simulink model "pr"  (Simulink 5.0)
settings: Solver=ode45  StartTime=0.0  StopTime=2  RelTol=1e-3
undefined symbols (not defined in the file or in its folder): sigbuilder_block
libraries: simulink x6

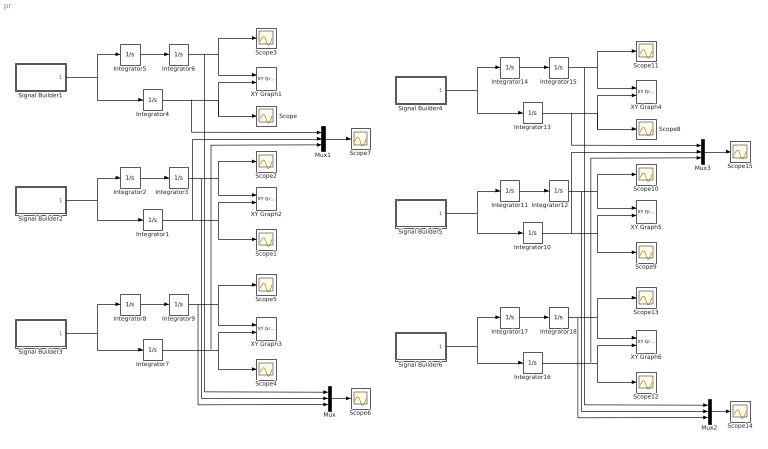
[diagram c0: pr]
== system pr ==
  Integrator{1..18} (18 alike) : Integrator
  Mux{,1..3} (4 alike) : Mux  Inputs=3
  Scope{,1..15} (16 alike) : Scope
  Signal Builder1 : Subsystem  Tag=STV Subsys  StartFcn=sigbuilder_block('start');  StopFcn=sigbuilder_block('stop');  ClipboardFcn=sigbuilder_block('clipboard');
  Signal Builder2 : Subsystem  Tag=STV Subsys  StartFcn=sigbuilder_block('start');  StopFcn=sigbuilder_block('stop');  ClipboardFcn=sigbuilder_block('clipboard');
  Signal Builder3 : Subsystem  Tag=STV Subsys  StartFcn=sigbuilder_block('start');  StopFcn=sigbuilder_block('stop');  ClipboardFcn=sigbuilder_block('clipboard');
  Signal Builder4 : Subsystem  Tag=STV Subsys  StartFcn=sigbuilder_block('start');  StopFcn=sigbuilder_block('stop');  ClipboardFcn=sigbuilder_block('clipboard');
  Signal Builder5 : Subsystem  Tag=STV Subsys  StartFcn=sigbuilder_block('start');  StopFcn=sigbuilder_block('stop');  ClipboardFcn=sigbuilder_block('clipboard');
  Signal Builder6 : Subsystem  Tag=STV Subsys  StartFcn=sigbuilder_block('start');  StopFcn=sigbuilder_block('stop');  ClipboardFcn=sigbuilder_block('clipboard');
  XY Graph1 : simulink/Sinks/XY Graph  xmin=0  xmax=3.5  ymin=0  ymax=3.5  st=-1
  XY Graph2 : simulink/Sinks/XY Graph  xmin=0  xmax=3.5  ymin=0  ymax=3.5  st=-1
  XY Graph3 : simulink/Sinks/XY Graph  xmin=0  xmax=3.5  ymin=0  ymax=3.5  st=-1
  XY Graph4 : simulink/Sinks/XY Graph  xmin=-4  xmax=0  ymin=-4  ymax=1.5  st=-1
  XY Graph5 : simulink/Sinks/XY Graph  xmin=-4  xmax=0  ymin=-4  ymax=1.5  st=-1
  XY Graph6 : simulink/Sinks/XY Graph  xmin=-4  xmax=0  ymin=-4  ymax=1.5  st=-1
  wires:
  Signal Builder1/1(Signal 2) -> Integrator4/1, Integrator5/1
  Integrator5/1 -> Integrator6/1
  Integrator6/1 -> XY Graph1/1, Scope3/1, Mux/1
  Integrator4/1 -> XY Graph1/2, Scope/1, Mux1/1
  Signal Builder2/1(Signal 2) -> Integrator1/1, Integrator2/1
  Integrator2/1 -> Integrator3/1
  Integrator3/1 -> XY Graph2/1, Scope2/1, Mux/2
  Integrator1/1 -> XY Graph2/2, Scope1/1, Mux1/2
  Signal Builder3/1(Signal 3) -> Integrator7/1, Integrator8/1
  Integrator8/1 -> Integrator9/1
  Integrator9/1 -> XY Graph3/1, Scope5/1, Mux/3
  Integrator7/1 -> XY Graph3/2, Scope4/1, Mux1/3
  Mux1/1 -> Scope7/1
  Mux/1 -> Scope6/1
  Signal Builder4/1(Signal 2) -> Integrator13/1, Integrator14/1
  Integrator14/1 -> Integrator15/1
  Integrator15/1 -> XY Graph4/1, Scope11/1, Mux2/1
  Integrator13/1 -> XY Graph4/2, Scope8/1, Mux3/1
  Signal Builder5/1(Signal 2) -> Integrator10/1, Integrator11/1
  Integrator11/1 -> Integrator12/1
  Integrator12/1 -> XY Graph5/1, Scope10/1, Mux2/2
  Integrator10/1 -> XY Graph5/2, Scope9/1, Mux3/2
  Signal Builder6/1(Signal 3) -> Integrator16/1, Integrator17/1
  Integrator17/1 -> Integrator18/1
  Integrator18/1 -> XY Graph6/1, Scope13/1, Mux2/3
  Integrator16/1 -> XY Graph6/2, Scope12/1, Mux3/3
  Mux3/1 -> Scope15/1
  Mux2/1 -> Scope14/1

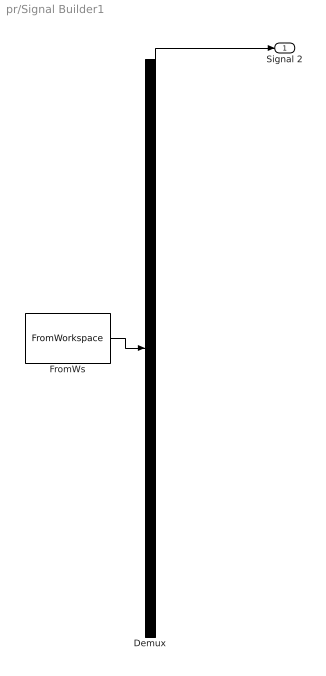
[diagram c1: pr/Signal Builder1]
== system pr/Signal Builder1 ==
  Demux : Demux  Tag=STV Demux  Outputs=1
  FromWs : FromWorkspace  Tag=STV FromWs  VariableName=tuvar  SampleTime=0  SigBuilderData=DataTag0
  Signal 2 : Outport  Tag=STV Outport
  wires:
  FromWs/1 -> Demux/1
  Demux/1 -> Signal 2/1

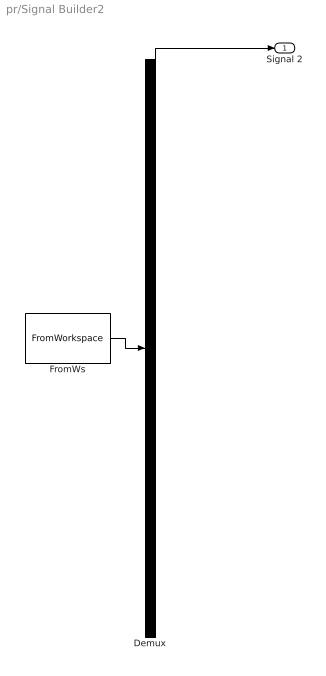
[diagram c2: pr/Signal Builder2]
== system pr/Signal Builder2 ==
  Demux : Demux  Tag=STV Demux  Outputs=1
  FromWs : FromWorkspace  Tag=STV FromWs  VariableName=tuvar  SampleTime=0  SigBuilderData=DataTag1
  Signal 2 : Outport  Tag=STV Outport
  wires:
  FromWs/1 -> Demux/1
  Demux/1 -> Signal 2/1

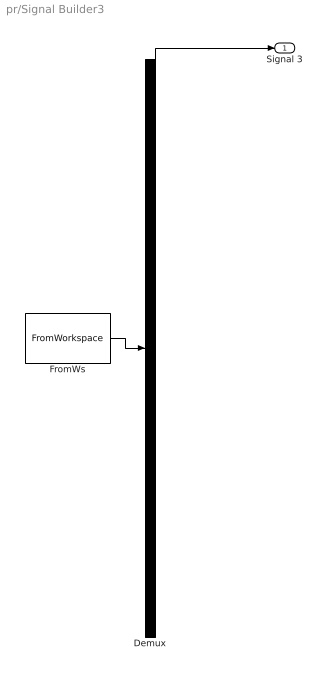
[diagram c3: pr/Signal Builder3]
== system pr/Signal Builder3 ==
  Demux : Demux  Tag=STV Demux  Outputs=1
  FromWs : FromWorkspace  Tag=STV FromWs  VariableName=tuvar  SampleTime=0  SigBuilderData=DataTag2
  Signal 3 : Outport  Tag=STV Outport
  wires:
  FromWs/1 -> Demux/1
  Demux/1 -> Signal 3/1

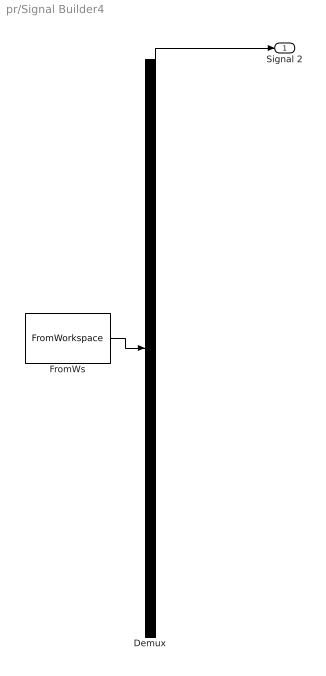
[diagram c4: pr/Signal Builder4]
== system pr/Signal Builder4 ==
  Demux : Demux  Tag=STV Demux  Outputs=1
  FromWs : FromWorkspace  Tag=STV FromWs  VariableName=tuvar  SampleTime=0  SigBuilderData=DataTag3
  Signal 2 : Outport  Tag=STV Outport
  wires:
  FromWs/1 -> Demux/1
  Demux/1 -> Signal 2/1

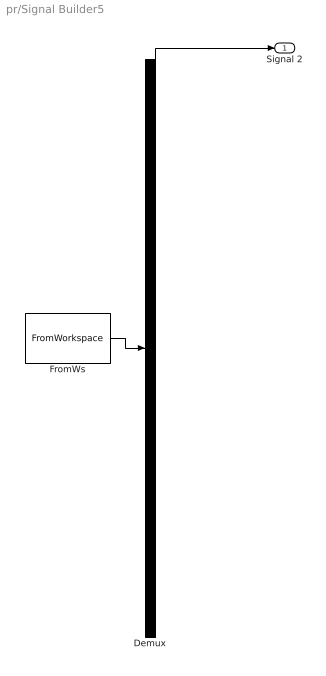
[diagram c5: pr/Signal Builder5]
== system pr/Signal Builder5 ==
  Demux : Demux  Tag=STV Demux  Outputs=1
  FromWs : FromWorkspace  Tag=STV FromWs  VariableName=tuvar  SampleTime=0  SigBuilderData=DataTag4
  Signal 2 : Outport  Tag=STV Outport
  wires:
  FromWs/1 -> Demux/1
  Demux/1 -> Signal 2/1

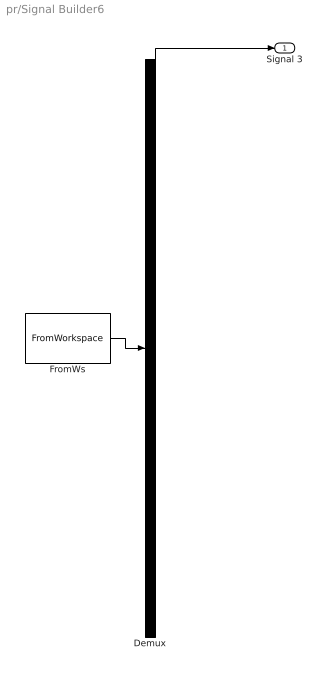
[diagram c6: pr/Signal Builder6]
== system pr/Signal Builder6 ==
  Demux : Demux  Tag=STV Demux  Outputs=1
  FromWs : FromWorkspace  Tag=STV FromWs  VariableName=tuvar  SampleTime=0  SigBuilderData=DataTag5
  Signal 3 : Outport  Tag=STV Outport
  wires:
  FromWs/1 -> Demux/1
  Demux/1 -> Signal 3/1
